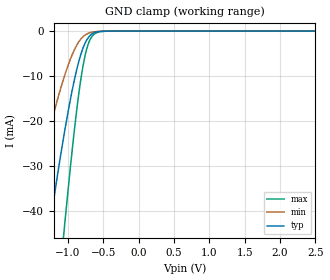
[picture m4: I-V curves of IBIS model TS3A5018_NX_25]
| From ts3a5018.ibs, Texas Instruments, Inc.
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[Model]   TS3A5018_NX_25
Model_type  Terminator
| variable   typ   min   max
C_comp   3.87pF   3.42pF   4.27pF
| C_tri-state   3.87pF   3.42pF   4.27pF
[Temperature Range]   40   100   -40
| Ambient temperature   25   85   -40
[Voltage range]   2.5   2.3   2.7
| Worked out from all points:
|   GND clamp passes 1 mA (typ) near -0.69 V on its own axis
[GND Clamp]
| TS3A5018_NX_25
|   Voltage   I(typ)   I(min)   I(max)
-2.5V     -224.8mA   -139mA     -345.3mA
-1.58V    -83.02mA   -45.6mA    -141.4mA
-1.555V   -79.7mA    -43.54mA   -136.4mA
-1.26V    -43.84mA   -21.95mA   -79.71mA
-1.06V    -23.45mA   -10.52mA   -45.18mA
-950mV    -13.93mA   -5.632mA   -27.88mA
-865mV    -7.852mA   -2.845mA   -16.14mA
-800mV    -4.324mA   -1.449mA   -8.938mA
-745mV    -2.269mA   -750.1uA   -4.58mA
-660mV    -630.3uA   -257.3uA   -1.201mA
-515mV    -41.74uA   -28.07uA   -88.02uA
2.5V      1.821nA    70.66pA    19.35nA
